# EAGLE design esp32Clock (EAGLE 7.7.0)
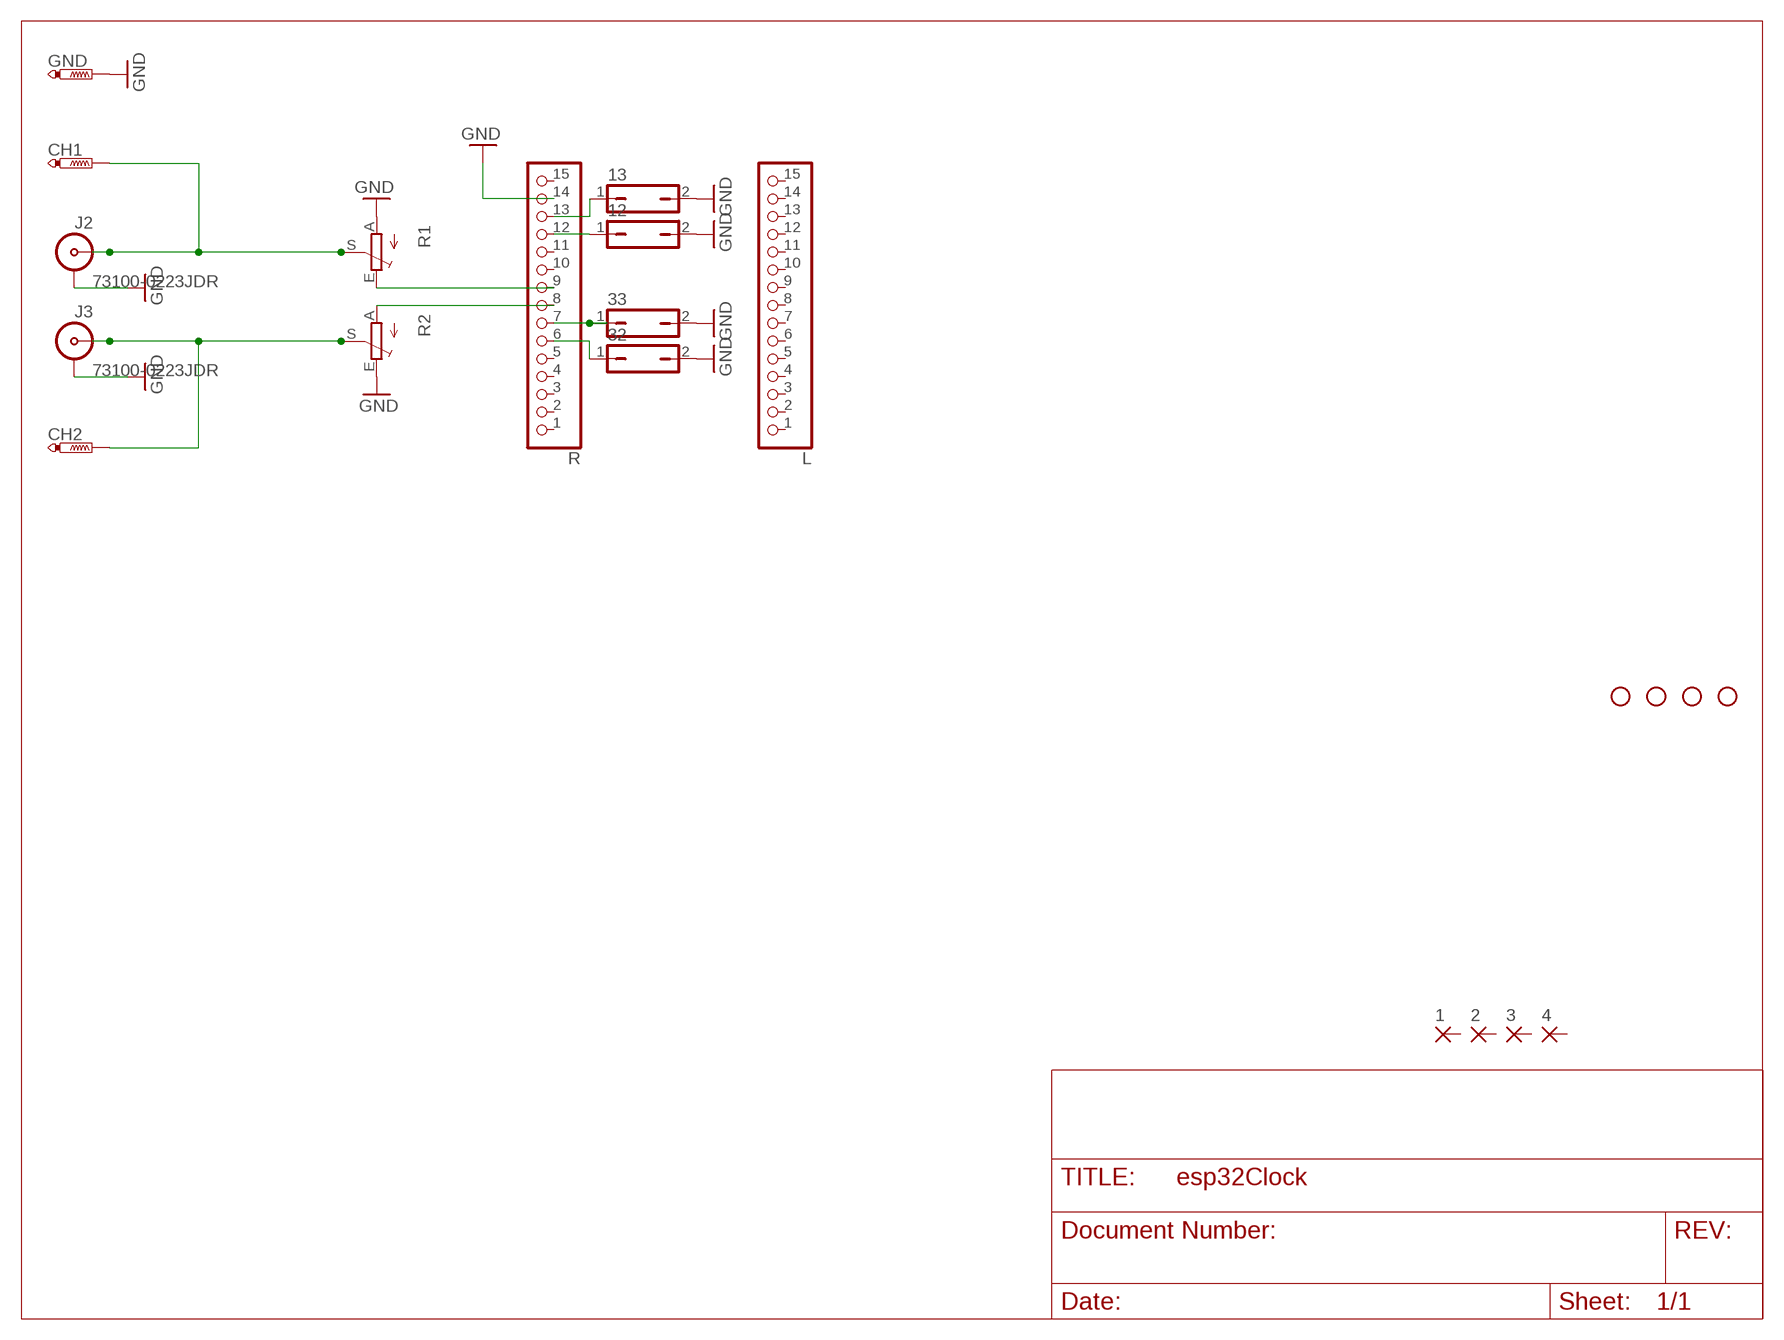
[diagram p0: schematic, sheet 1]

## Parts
1  3,17/1,1  [3,17/1,1]
2  3,17/1,1  [3,17/1,1]
3  3,17/1,1  [3,17/1,1]
4  3,17/1,1  [3,17/1,1]
12  JP1Q  [JP1]
13  JP1Q  [JP1]
32  JP1Q  [JP1]
33  JP1Q  [JP1]
CH1  PTR1PAD1-20Y  [P1-20Y]
CH2  PTR1PAD1-20Y  [P1-20Y]
GND  PTR1PAD1-20Y  [P1-20Y]
J2  73100-0223JDR  [73100-0223JDR]
J3  73100-0223JDR  [73100-0223JDR]
L  PINHD-1X15  [1X15]
R  PINHD-1X15  [1X15]
R1  TRIM_EU-CA6V  [CA6V]
R2  TRIM_EU-CA6V  [CA6V]
U$2  STAND-OFF  [STAND-OFF]
U$3  STAND-OFF  [STAND-OFF]
U$4  STAND-OFF  [STAND-OFF]
U$5  STAND-OFF  [STAND-OFF]

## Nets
GND: 12.2 13.2 32.2 33.2 GND.1(TP) J2.GND J3.GND R1.A R2.E R.14
N$1: 33.1 R.7
N$2: 32.1 R.6
N$3: 12.1 R.12
N$4: 13.1 R.13
N$5: CH1.1(TP) J2.P R1.S
N$6: R1.E R.9
N$7: CH2.1(TP) J3.P R2.S
N$8: R2.A R.8
Unconnected: 1.1(P) 2.1(P) 3.1(P) 4.1(P) L.1 L.2 L.3 L.4 L.5 L.6 L.7 L.8 L.9 L.10 L.11 L.12 L.13 L.14 L.15 R.1 R.2 R.3 R.4 R.5 R.10 R.11 R.15

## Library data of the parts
1-4 = wirepad:3,17/1,1: THROUGH-HOLE PAD
12 13 32 33 = jumper:JP1Q: JUMPER
CH1 CH2 GND = testpad:PTR1: TEST PIN
J2 J3 = con-coax:73100-0223: BNC CONNECTOR - Molex
L R = pinhead:PINHD-1X15: PIN HEADER
R1 R2 = pot:TRIM_EU-: POTENTIOMETER
U$2-U$5 = SparkFun:STAND-OFF: Stand Off

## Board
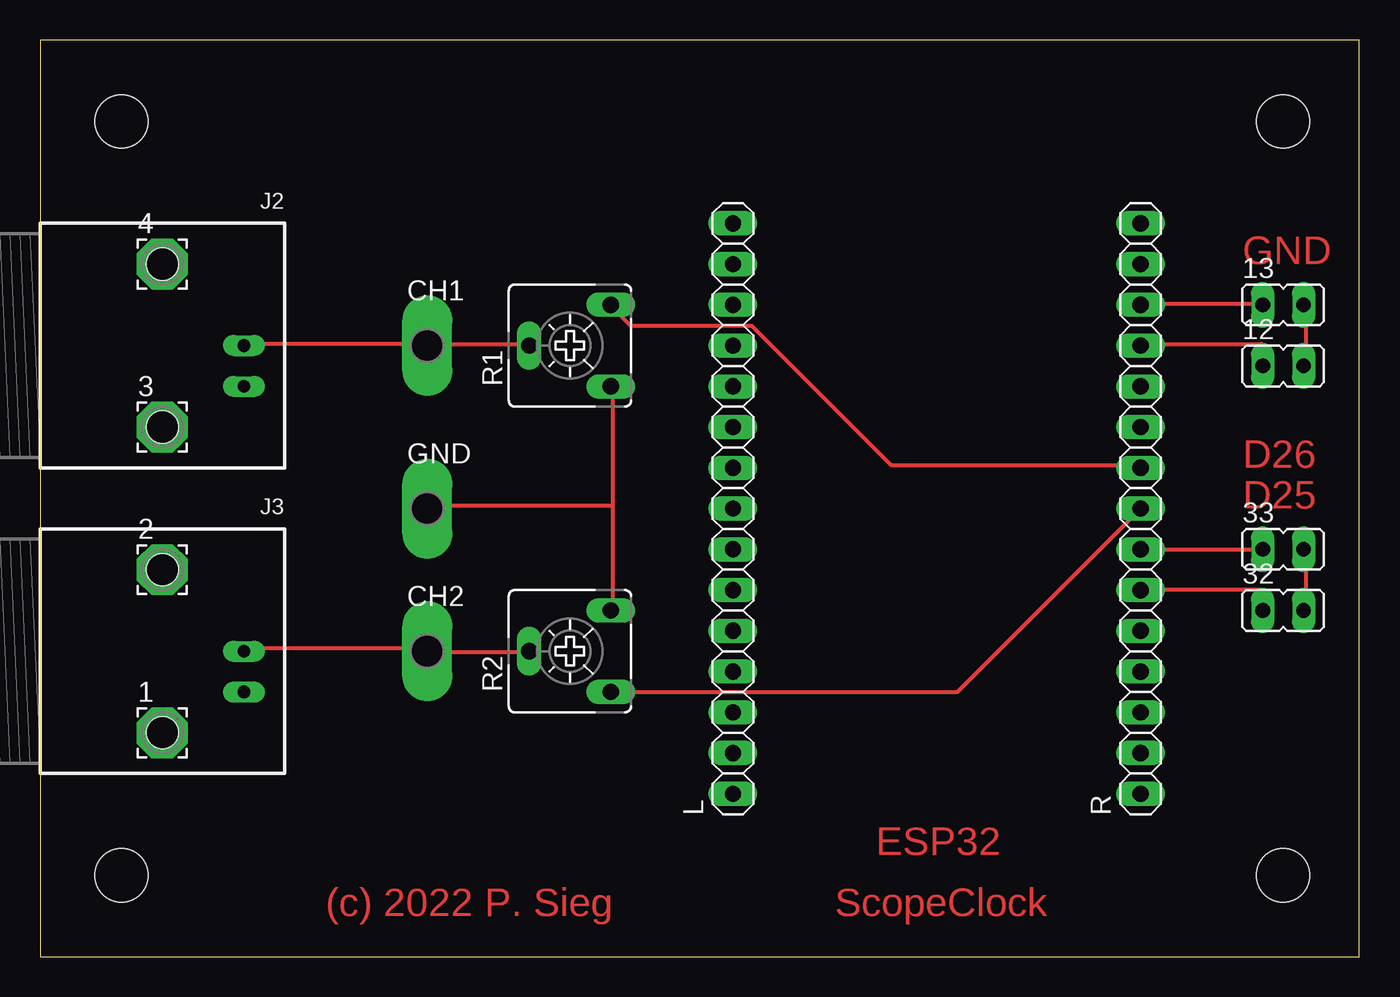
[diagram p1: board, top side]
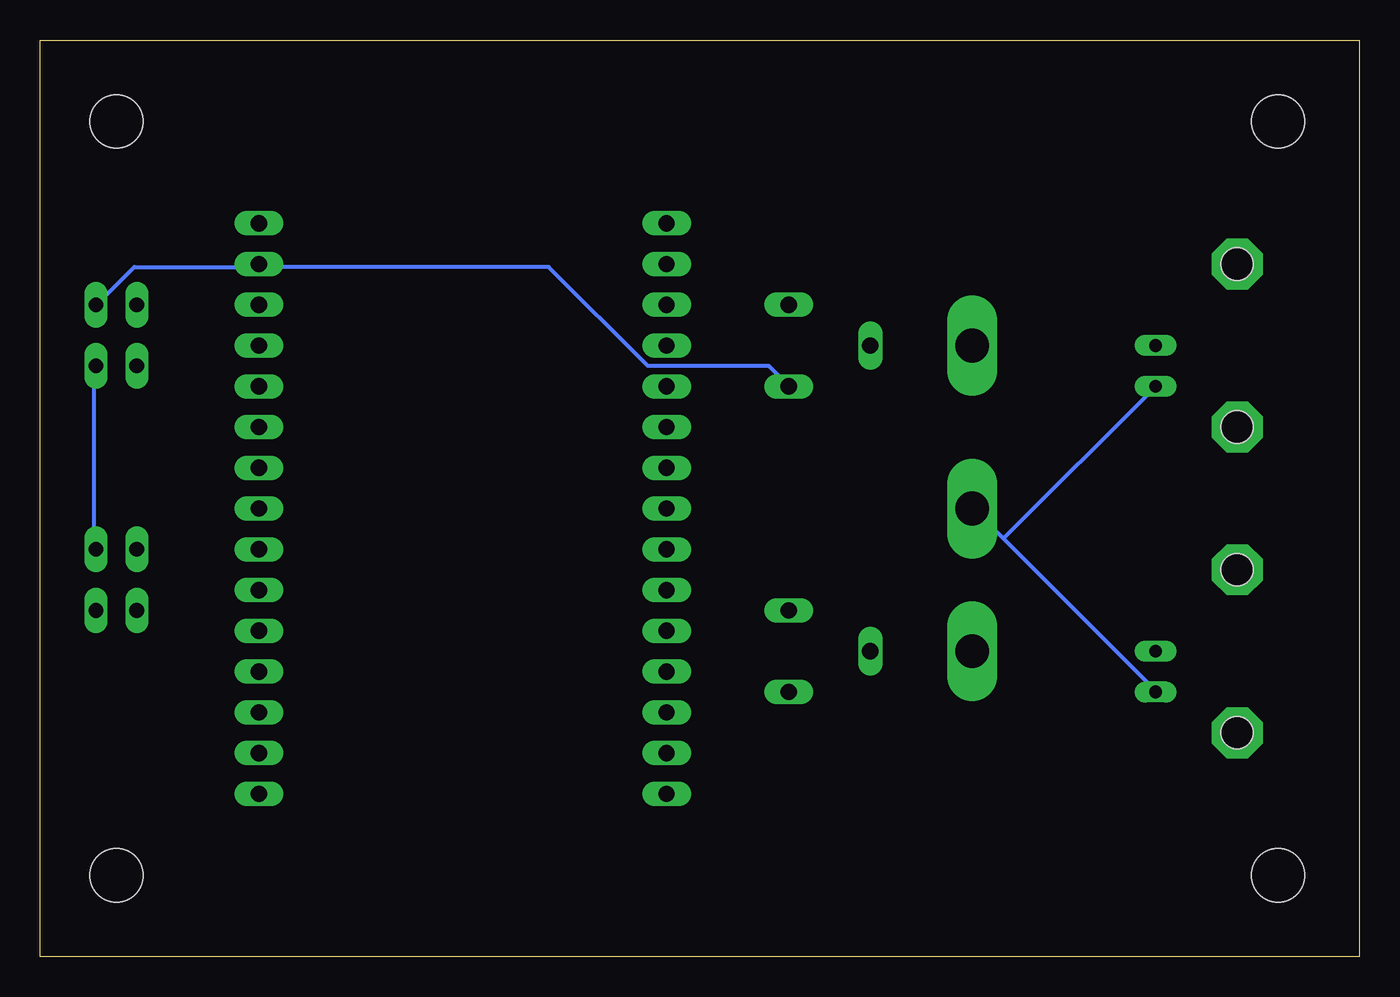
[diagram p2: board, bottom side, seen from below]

Size 82.22 x 57.14 mm. Coordinates in mm from the lower left corner, seen from the top.
Outline: 0,0 82.22,0 82.22,57.14 0,57.14 0,0
Copper layers (1*16): Top 0.035mm / dielectric 1.5mm / Bottom 0.035mm
Design rules "default": minimum track width 10mil, minimum drill 24mil, track to track 8mil, track to pad 8mil, pad to pad 8mil, via to via 8mil, smd to smd 8mil, copper to edge 40mil, drill to drill 8mil, minimum pad ring 10mil, minimum via ring 8mil, stop-mask expansion 4mil, vias tented up to drill 0mil, thermal gap 10mil

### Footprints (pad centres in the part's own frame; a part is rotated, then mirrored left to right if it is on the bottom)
3,17/1,1 = drill 1.118 pad 3.175 octagon: 1 0,0
JP1 = drill 0.914 long: 1 0,-1.27; 2 0,1.27
P1-20Y = drill 2.1 pad 2.54 long: 1 0,0
73100-0223JDR = drill 0.8 long: GND 0,-2.54; P 0,0 | hole 2.007: -5.08,-5.08; -5.08,5.08
1X15 = drill 1.016 long: 1 -17.78,0; 2 -15.24,0; 3 -12.7,0; 4 -10.16,0; 5 -7.62,0; 6 -5.08,0; 7 -2.54,0; 8 0,0; 9 2.54,0; 10 5.08,0; 11 7.62,0; 12 10.16,0; 13 12.7,0; 14 15.24,0; 15 17.78,0
CA6V = drill 1.016 long: A -2.54,-2.54; E 2.54,-2.54; S 0,2.54
STAND-OFF = hole 3.302: 0,0

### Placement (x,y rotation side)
1  7.62,13.97 0 top
2  7.62,24.13 0 top
3  7.62,33.02 0 top
4  7.62,43.18 0 top
12  77.47,36.83 270 top
13  77.47,40.64 270 top
32  77.47,21.59 270 top
33  77.47,25.4 270 top
CH1  24.13,38.1 0 top
CH2  24.13,19.05 0 top
GND  24.13,27.94 0 top
J2  12.7,38.1 0 top
J3  12.7,19.05 0 top
L  43.18,27.94 90 top
R  68.58,27.94 90 top
R1  33.02,38.1 90 top
R2  33.02,19.05 90 top
U$2  77.47,5.08 0 top
U$3  5.08,5.08 0 top
U$4  77.47,52.07 0 top
U$5  5.08,52.07 0 top

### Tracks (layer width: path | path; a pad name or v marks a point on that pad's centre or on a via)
GND
  Top 0.254: 32.2 78.87,22.88 78.87,25.4 33.2 | 12.2 78.87,38.2 78.87,40.49 13.2 | 35.66,28.14 35.66,35.46 R1.A | 35.66,28.14 35.66,21.74 R2.E | 35.66,28.14 24.23,28.14 GND.1
  Bottom 0.254: 68.58,43 76.35,43 78.64,40.72 13.2 | 33.2 78.87,25.4 78.87,37.97 12.2 | 22.17,26.09 24,27.91 GND.1 | 22.17,26.09 12.8,16.71 J3.GND | 22.17,26.09 J2.GND | 68.58,43 50.52,43 44.35,36.83 36.8,36.83 35.66,35.69 R1.A | 68.58,43 R.14
N$1
  Top 0.254: R.7 33.1
N$2
  Top 0.254: 32.1 76.12,22.88 68.58,22.88 R.6
N$3
  Top 0.254: 12.1 76.12,38.2 68.58,38.2 R.12
N$4
  Top 0.254: 13.1 76.12,40.72 68.58,40.72 R.13
N$5
  Top 0.254: J2.P 12.8,38.2 24,38.2 CH1.1 24.23,38.2 30.4,38.2 R1.S
N$6
  Top 0.254: R.9 68.58,30.66 53.03,30.66 44.35,39.34 36.8,39.34 35.66,40.49 R1.E
N$7
  Top 0.254: J3.P 12.8,19.23 24,19.23 CH2.1 24.23,19 30.4,19 R2.S
N$8
  Top 0.254: R2.A 35.66,16.48 57.15,16.48 68.58,27.91 R.8

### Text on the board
Top: GND | D26 | D25 | ESP32 | (c) 2022 P. Sieg | ScopeClock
